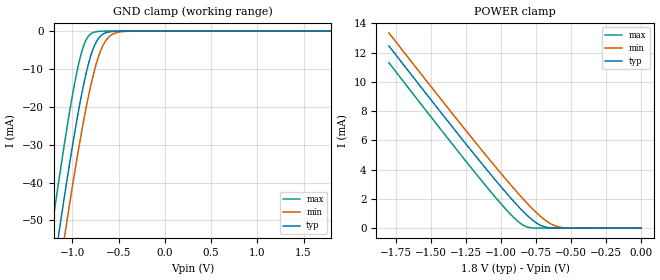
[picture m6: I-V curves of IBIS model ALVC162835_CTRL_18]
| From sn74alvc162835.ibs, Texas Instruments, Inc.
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[Model]   ALVC162835_CTRL_18
Model_type  Input
Vinl=0.5775
Vinh=1.2675
| variable   typ   min   max
C_comp   11.50pF   11.13pF   11.64pF
[Temperature Range]   40   100   -40
| Ambient temperature   25   85   -40
[Voltage range]   1.8   1.65   1.95
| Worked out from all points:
|   GND clamp passes 1 mA (typ) near -0.68 V on its own axis
|   POWER clamp passes 1 mA (typ) near -0.83 V on its own axis
[GND Clamp]
| ALVC162835_CTRL_18
|   Voltage   I(typ)   I(min)   I(max)
-1.8V     -169.5mA   -179.7mA   -156.7mA
-1.245V   -70.18mA   -81.02mA   -56.25mA
-1.22V    -65.92mA   -76.78mA   -51.96mA
-1.14V    -52.55mA   -63.42mA   -38.55mA
-1.075V   -42.06mA   -52.87mA   -28.16mA
-920mV    -19.37mA   -29.44mA   -7.486mA
-860mV    -12.16mA   -21.41mA   -2.808mA
-795mV    -6.112mA   -13.8mA    -645.2uA
-730mV    -2.404mA   -7.745mA   -117.8uA
-660mV    -692.8uA   -3.428mA   -17.66uA
-495mV    -25.94uA   -270.9uA   -195.5nA
1.8V      1.111nA    59.78nA    3.14pA
[POWER Clamp]
| ALVC162835_CTRL_18
|   Voltage   I(typ)   I(min)   I(max)
-1.8V     12.46mA    13.35mA    11.31mA
-1.385V   7.377mA    8.289mA    6.203mA
-1.11V    4.096mA    5.012mA    2.913mA
-945mV    2.219mA    3.118mA    1.08mA
-890mV    1.63mA     2.511mA    555.9uA
-850mV    1.223mA    2.082mA    253.5uA
-800mV    757.1uA    1.566mA    48.87uA
-720mV    203.3uA    821.4uA    1.201uA
-655mV    31.58uA    351.6uA    51.18nA
-595mV    3.897uA    103.1uA    2.775nA
-490mV    89.19nA    5.424uA    22.18pA
-16.28fV  1.111nA    59.61nA    3.661pA
